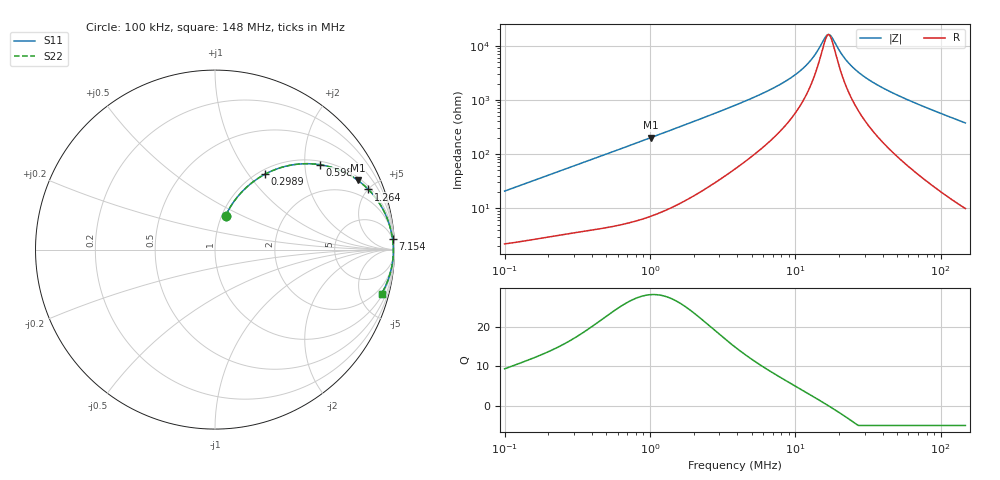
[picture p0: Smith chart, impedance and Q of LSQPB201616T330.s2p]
! LSQPB201616T330  S-PARAMETER MODEL  ( General Type )
! Model Generated by TAIYO YUDEN Corporation (http://www.ty-top.com)
! Version 2.0
! TAIYO YUDEN Control No. 100810NC14SB-FKC
! Copyright(c) 2008 TAIYO YUDEN CO.,LTD. All Rights Reserved.
! Product Description (link to TY-COMPAS)
! https://ds.yuden.co.jp/TYCOMPAS/or/detail?pn=LSQPB201616T330K&u=M
! Products Name : Inductors
! Characteristics :
!  Inductance : 33 uH , SRF(min) : 13 MHz , DC Resistance(max) : 2.21 Ohm
!  Rated Current : Saturation :270 mA , Temp Rise : 240 mA (40 degC)
!  Case Size : 2.0 x 1.6 / 0.079 x 0.063 [mm/inch] , Thickness : 1.6 / 0.063 [mm/inch]
!  (Conditions: Temperature = 25 degC , DC Bias Current/Voltage = 0A / 0V)
! External Node Assignments :
!  1  o---GGG---o  2
! GND o---------o GND
! Frequency Range : 0.1MHz  -  147.97148MHz  [ 402 STEP ]
# MHz S RI R 50
! Freq[MHz].  S11 Real  S11 Imag  S21 Real  S21 Imag  S12 Real  S12 Imag  S22 Real  S22 Imag
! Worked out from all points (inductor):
!   401 points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, 100 kHz to 148 MHz, reference 50 ohm
!   read as one part in series: L = 32.7 uH near 103.7 kHz
!   highest Q = 28.3 at 1.015 MHz (marker M1), where L = 31.6 uH
!   self-resonance near 16.87 MHz
!   S11 on the Smith chart (normalised r, x): 100 kHz: 1.04, +0.41; 298.9 kHz: 1.07, +1.20; 598 kHz: 1.10, +2.38; 1.264 MHz: 1.18, +5.02; 7.154 MHz: 5, +33; 148 MHz: 1.20, -7.51
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0.1  0.0598 0.1898  0.9402 -0.1898  0.9402 -0.1898  0.0598 0.1898
0.179314  0.1362 0.3066  0.8638 -0.3066  0.8638 -0.3066  0.1362 0.3066
0.298901  0.2771 0.4193  0.7229 -0.4193  0.7229 -0.4193  0.2771 0.4193
0.339629  0.3259 0.4423  0.6741 -0.4423  0.6741 -0.4423  0.3259 0.4423
0.59799  0.5828 0.4733  0.4172 -0.4733  0.4172 -0.4733  0.5828 0.4733
1.015153  0.7943 0.3869  0.2057 -0.3869  0.2057 -0.3869  0.7943 0.3869
1.153479  0.8315 0.357  0.1685 -0.357  0.1685 -0.357  0.8315 0.357
1.263679  0.8545 0.3351  0.1455 -0.3351  0.1455 -0.3351  0.8545 0.3351
2.068349  0.9363 0.2236  0.0637 -0.2236  0.0637 -0.2236  0.9363 0.2236
3.917549  0.9772 0.1192  0.0228 -0.1192  0.0228 -0.1192  0.9772 0.1192
7.154086  0.9894 0.0579  0.0106 -0.0579  0.0106 -0.0579  0.9894 0.0579
10.30536  0.9924 0.0311  0.00761 -0.0311  0.00761 -0.0311  0.9924 0.0311
13.06453  0.9934 0.0158  0.00662 -0.0158  0.00662 -0.0158  0.9934 0.0158
15.96885  0.9938 0.00349  0.00621 -0.00349  0.00621 -0.00349  0.9938 0.00349
17.17811  0.9939 -0.000936  0.00614 0.000936  0.00614 0.000936  0.9939 -0.000936
18.14478  0.9939 -0.00426  0.00613 0.00426  0.00613 0.00426  0.9939 -0.00426
21.3836  0.9938 -0.0144  0.00623 0.0144  0.00623 0.0144  0.9938 -0.0144
25.20054  0.9934 -0.0249  0.00658 0.0249  0.00658 0.0249  0.9934 -0.0249
31.94778  0.9924 -0.0413  0.00763 0.0413  0.00763 0.0413  0.9924 -0.0413
44.37094  0.9894 -0.0679  0.0106 0.0679  0.0106 0.0679  0.9894 -0.0679
76.71177  0.9769 -0.1291  0.0231 0.1291  0.0231 0.1291  0.9769 -0.1291
147.9715  0.9283 -0.2452  0.0717 0.2452  0.0717 0.2452  0.9283 -0.2452
